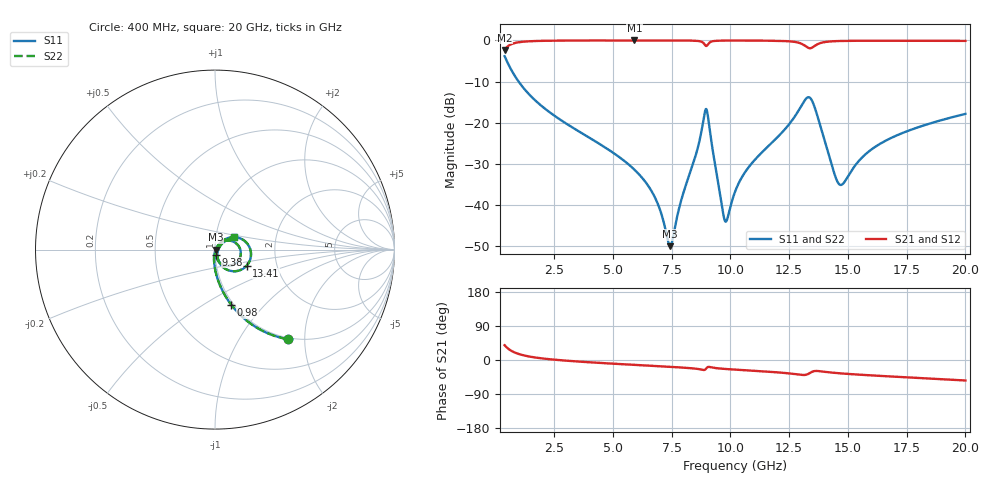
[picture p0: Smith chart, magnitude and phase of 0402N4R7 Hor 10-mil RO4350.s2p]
# MHz S  dB  R 50
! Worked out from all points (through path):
!   1961 points, 400 MHz to 20 GHz, reference 50 ohm
!   highest |S21| = -0.02 dB at 5.92 GHz (marker M1); lowest = -2.3 dB at 400 MHz (marker M2)
!   group delay of S21, straight-line fit = 9.04 ps
!   lowest |S11| = -50.0 dB at 7.44 GHz (marker M3), VSWR 1.01, Z = 50.3 - j0.121 ohm
!   |S11| at or under -10 dB: 994.6 MHz to end of sweep
!   |S22| runs from -50.0 to -3.8 dB; largest |S21 - S12| = 0
!   S11 on the Smith chart (normalised r, x): 400 MHz: 0.97, -1.65; 980 MHz: 0.97, -0.67; 9.38 GHz: 1.01, -0.06; 13.41 GHz: 1.40, -0.26; 20 GHz: 1.23, +0.17
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400  -3.85 -51.0  -2.31 39.0  -2.31 39.0  -3.85 -51.0
980  -9.88 -73.6  -0.48 16.3  -0.48 16.3  -9.88 -73.6
2000  -16.06 -85.4  -0.12 4.2  -0.12 4.2  -16.06 -85.4
3670  -22.50 -93.4  -0.04 -4.7  -0.04 -4.7  -22.50 -93.4
5920  -31.39 -97.9  -0.03 -12.9  -0.03 -12.9  -31.39 -97.9
6940  -40.05 -90.2  -0.03 -16.3  -0.03 -16.3  -40.05 -90.2
7440  -49.98 -22.2  -0.03 -18.0  -0.03 -18.0  -49.98 -22.2
8590  -26.68 50.3  -0.13 -23.4  -0.13 -23.4  -26.68 50.3
8940  -16.93 -1.9  -1.24 -24.8  -1.24 -24.8  -16.93 -1.9
9050  -18.49 -49.5  -0.96 -18.4  -0.96 -18.4  -18.49 -49.5
9380  -31.11 -82.3  -0.12 -21.3  -0.12 -21.3  -31.11 -82.3
9780  -43.92 -24.6  -0.06 -23.6  -0.06 -23.6  -43.92 -24.6
10200  -36.80 43.6  -0.05 -25.4  -0.05 -25.4  -36.80 43.6
10810  -30.59 52.0  -0.05 -27.7  -0.05 -27.7  -30.59 52.0
12870  -17.36 30.5  -0.52 -38.1  -0.52 -38.1  -17.36 30.5
13410  -14.07 -26.8  -1.91 -33.4  -1.91 -33.4  -14.07 -26.8
13470  -14.59 -35.9  -1.79 -31.4  -1.79 -31.4  -14.59 -35.9
13870  -21.54 -70.2  -0.59 -30.0  -0.59 -30.0  -21.54 -70.2
14660  -35.06 -22.2  -0.16 -35.2  -0.16 -35.2  -35.06 -22.2
15710  -27.87 37.5  -0.09 -39.6  -0.09 -39.6  -27.87 37.5
16740  -23.98 40.3  -0.09 -43.2  -0.09 -43.2  -23.98 40.3
20000  -17.85 33.1  -0.13 -54.1  -0.13 -54.1  -17.85 33.1
